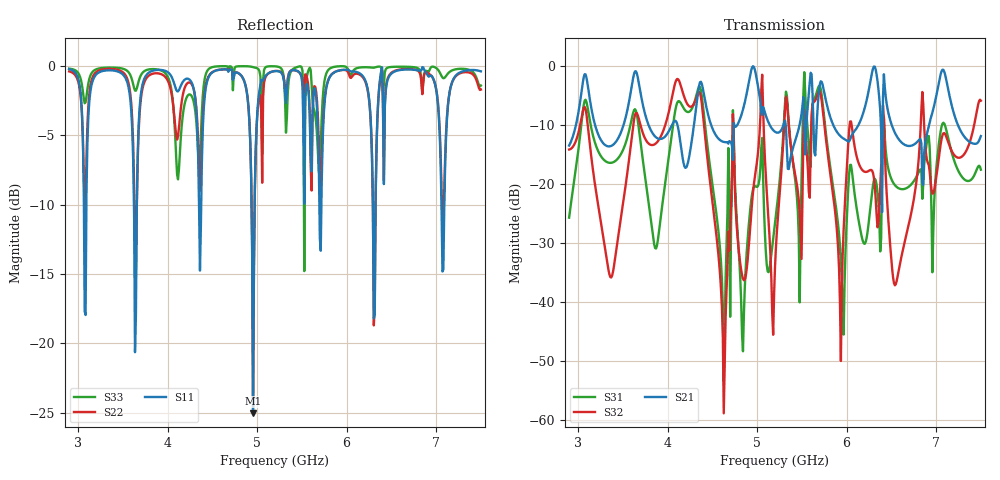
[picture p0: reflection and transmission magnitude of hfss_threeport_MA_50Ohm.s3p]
! Touchstone file from project Project1
! Exported from HFSS 2017.1.0
# GHZ S MA R 50.000000
! Modal data exported
! Port[1] = 1:1
! Port[2] = 2:1
! Port[3] = 3:1
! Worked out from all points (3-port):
!   451 points, 2.9 GHz to 7.5 GHz, reference 50 ohm
!   strongest paths, dB at 2.9 GHz, 4.045 GHz, 5.2 GHz, 6.355 GHz, 7.5 GHz:
!     S21: -13.5, -10.1, -11.2, -3.9, -11.9
!     S32: -14.2, -5.6, -34.1, -26.8, -5.9
!     S31: -25.7, -11.8, -26.7, -23.2, -17.6
!   lowest |S11| = -25.0 dB at 4.955 GHz (marker M1), VSWR 1.12, Z = 44.9 - j1.58 ohm
!   |S11| at or under -10 dB: 3.624 GHz to 3.656 GHz (32.06 MHz wide, 0.881 % of centre); 4.938 GHz to 4.973 GHz (34.94 MHz wide, 0.705 % of centre); 7.059955 GHz to 7.091402 GHz (31.45 MHz wide, 0.444 % of centre)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
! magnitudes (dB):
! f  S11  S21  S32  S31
! 2.9 GHz  -0.2  -13.5  -14.2  -25.7
! 4.352 GHz  -10.1  -3.4  -4.4  -3.5
! 4.628 GHz  -0.2  -12.9  -58.8  -53.4
! 4.955 GHz  -25.0  0.0  -21.4  -20.9
! 5.2 GHz  -0.4  -11.2  -34.1  -26.7
! 5.323 GHz  -2.7  -10.3  -5.2  -4.4
! 5.936 GHz  -0.3  -12.0  -49.9  -32.7
! 6.048 GHz  -0.4  -12.0  -9.4  -16.7
! 6.549 GHz  -0.4  -11.6  -37.0  -20.3
! 7.5 GHz  -0.4  -11.9  -5.9  -17.6
